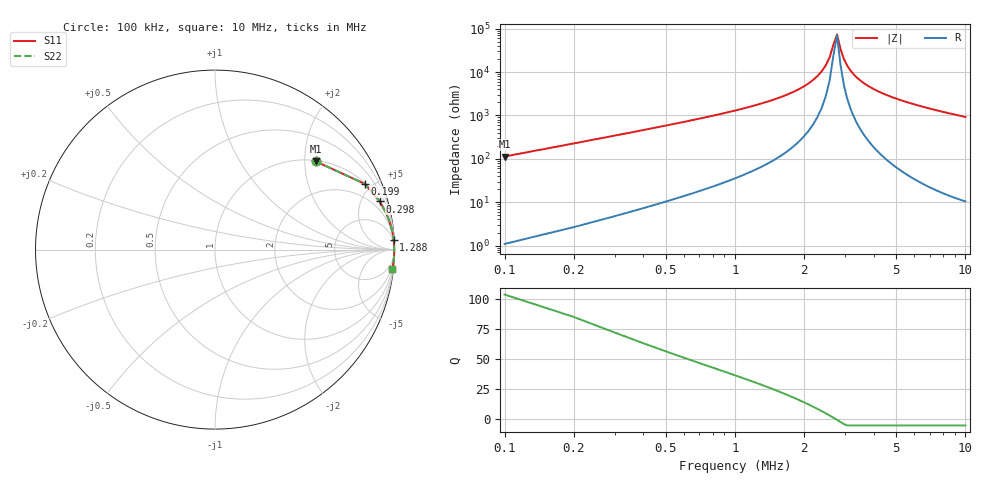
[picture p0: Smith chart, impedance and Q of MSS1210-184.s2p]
# MHz S MA R 50
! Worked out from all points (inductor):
!   101 points, 100 kHz to 10 MHz, reference 50 ohm
!   read as one part in series: L = 180 uH near 100 kHz
!   highest Q = 104 at 100 kHz (marker M1), where L = 180 uH
!   self-resonance near 2.674 MHz
!   S11 on the Smith chart (normalised r, x): 100 kHz: 1.02, +2.26; 199 kHz: 1.05, +4.52; 298 kHz: 1.09, +6.81; 1.288 MHz: 2, +37; 10 MHz: 1, -19
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0.1  0.746 41.2  0.6588 -48.2  0.6588 -48.2  0.746 41.2
0.199  0.9106 23.7  0.4027 -65.6  0.4027 -65.6  0.9106 23.7
0.298  0.956 16.3  0.2806 -72.9  0.2806 -72.9  0.956 16.3
0.496  0.9825 9.8  0.1697 -79.2  0.1697 -79.2  0.9825 9.8
0.694  0.9905 6.8  0.1184 -82.0  0.1184 -82.0  0.9905 6.8
1.288  0.9967 3.1  0.05361 -85.0  0.05361 -85.0  0.9967 3.1
1.783  0.998 1.7  0.02886 -85.2  0.02886 -85.2  0.998 1.7
2.08  0.9984 1.0  0.01834 -84.4  0.01834 -84.4  0.9984 1.0
2.377  0.9986 0.5  0.009608 -81.2  0.009608 -81.2  0.9986 0.5
2.575  0.9987 0.2  0.004535 -72.8  0.004535 -72.8  0.9987 0.2
2.674  0.9987 0.1  0.002312 -55.6  0.002312 -55.6  0.9987 0.1
2.773  0.9987 -0.0  0.001352 18.4  0.001352 18.4  0.9987 -0.0
2.872  0.9987 -0.2  0.002965 64.6  0.002965 64.6  0.9987 -0.2
2.971  0.9987 -0.3  0.005022 75.3  0.005022 75.3  0.9987 -0.3
3.07  0.9987 -0.4  0.007088 79.6  0.007088 79.6  0.9987 -0.4
3.268  0.9987 -0.6  0.0111 83.2  0.0111 83.2  0.9987 -0.6
3.466  0.9987 -0.9  0.01494 84.6  0.01494 84.6  0.9987 -0.9
4.06  0.9986 -1.5  0.02559 86.0  0.02559 86.0  0.9986 -1.5
5.05  0.9981 -2.4  0.04138 86.2  0.04138 86.2  0.9981 -2.4
6.733  0.9968 -3.7  0.0653 85.3  0.0653 85.3  0.9968 -3.7
8.416  0.9951 -5.0  0.08738 84.3  0.08738 84.3  0.9951 -5.0
10  0.993 -6.2  0.1072 83.2  0.1072 83.2  0.993 -6.2
